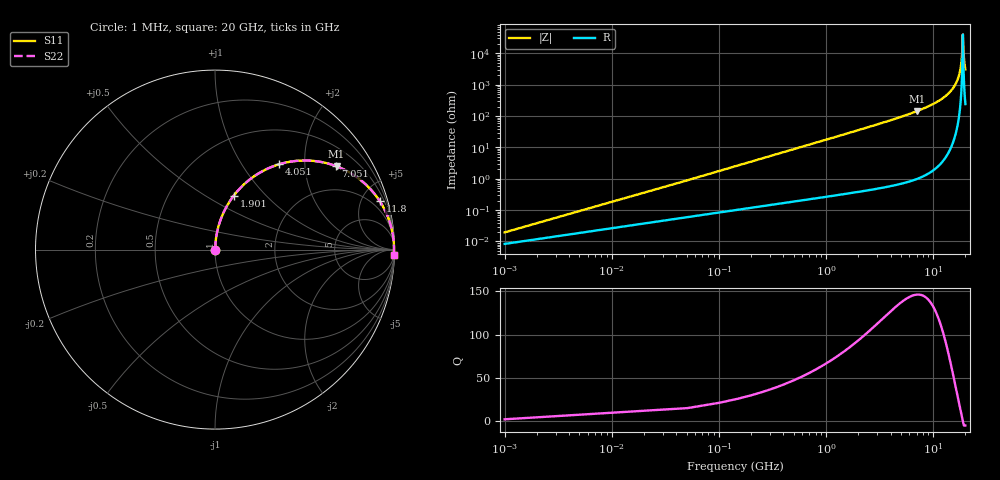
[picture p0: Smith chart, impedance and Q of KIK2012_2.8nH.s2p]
!version-2
!date-01.2022
!Series
# MHz S RI R 50
!Freq ReS11 ImS11 ReS21 ImS21 ReS12 ImS12 ReS22 ImS22
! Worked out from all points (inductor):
!   401 points, 1 MHz to 20 GHz, reference 50 ohm
!   read as one part in series: L = 2.8 nH near 101 MHz
!   highest Q = 146 at 7.101 GHz (marker M1), where L = 3.26 nH
!   self-resonance near 18.9 GHz
!   S11 on the Smith chart (normalised r, x): 1 MHz: 1.00, +0.00; 1.901 GHz: 1.01, +0.68; 4.051 GHz: 1.01, +1.49; 7.051 GHz: 1.02, +2.88; 11.8 GHz: 1.06, +6.78; 20 GHz: 6, -61
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1  8.35e-05 0.000176  0.9999 -0.000176  0.9999 -0.000176  8.35e-05 0.000176
151  0.00173 0.0265  0.9983 -0.0265  0.9983 -0.0265  0.00173 0.0265
251  0.00326 0.044  0.9967 -0.044  0.9967 -0.044  0.00326 0.044
351  0.00534 0.0613  0.9947 -0.0613  0.9947 -0.0613  0.00534 0.0613
901  0.0269 0.1542  0.9731 -0.1542  0.9731 -0.1542  0.0269 0.1542
1901  0.1051 0.3012  0.8949 -0.3012  0.8949 -0.3012  0.1051 0.3012
3351  0.272 0.4408  0.728 -0.4408  0.728 -0.4408  0.272 0.4408
4051  0.3591 0.4758  0.6409 -0.4758  0.6409 -0.4758  0.3591 0.4758
6701  0.6439 0.4754  0.3561 -0.4754  0.3561 -0.4754  0.6439 0.4754
7051  0.6735 0.4655  0.3265 -0.4655  0.3265 -0.4655  0.6735 0.4655
7101  0.6776 0.464  0.3224 -0.464  0.3224 -0.464  0.6776 0.464
10001  0.8542 0.3492  0.1458 -0.3492  0.1458 -0.3492  0.8542 0.3492
11801  0.918 0.2699  0.082 -0.2699  0.082 -0.2699  0.918 0.2699
13351  0.9539 0.204  0.0461 -0.204  0.0461 -0.204  0.9539 0.204
16701  0.9919 0.0752  0.00806 -0.0752  0.00806 -0.0752  0.9919 0.0752
17601  0.9957 0.044  0.00434 -0.044  0.00434 -0.044  0.9957 0.044
18201  0.997 0.024  0.00301 -0.024  0.00301 -0.024  0.997 0.024
18601  0.9974 0.0111  0.00257 -0.0111  0.00257 -0.0111  0.9974 0.0111
18851  0.9975 0.0031  0.00248 -0.0031  0.00248 -0.0031  0.9975 0.0031
18951  0.9975 -6.29e-05  0.00247 6.29e-05  0.00247 6.29e-05  0.9975 -6.29e-05
19401  0.9973 -0.0141  0.00271 0.0141  0.00271 0.0141  0.9973 -0.0141
20000  0.9964 -0.0322  0.0036 0.0322  0.0036 0.0322  0.9964 -0.0322
